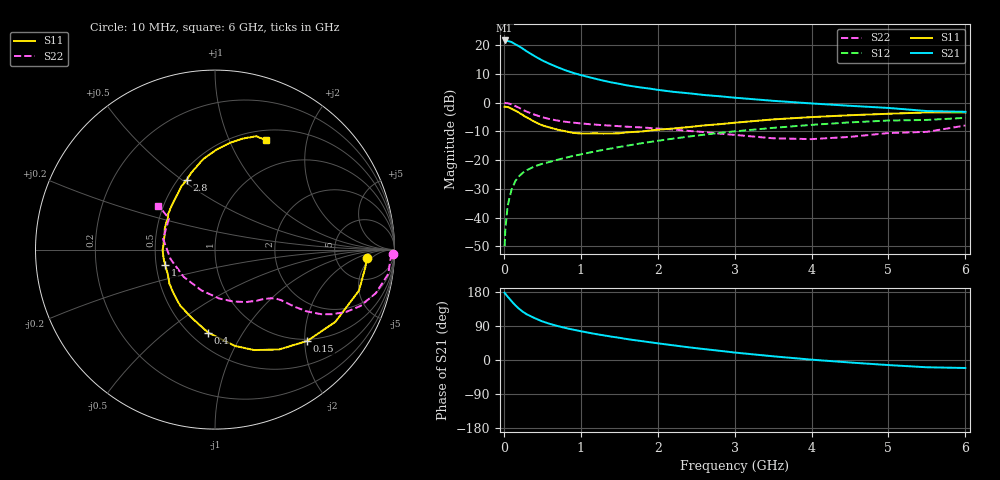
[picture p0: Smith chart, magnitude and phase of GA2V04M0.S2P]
! Infineon Technologies  Discrete & RF Semiconductors
! BF775
! Si NPN RF Bipolar Junction Transistor in SOT23
! VCE = 2 V  IC = 4 mA
! Common Emitter S-Parameters:  May  1996
# GHz  S  MA  R  50
!  f  S11  S21  S12  S22
! GHz  MAG  ANG  MAG  ANG  MAG  ANG  MAG  ANG
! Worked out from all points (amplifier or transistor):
!   36 points, 10 MHz to 6 GHz, reference 50 ohm
!   highest |S21| = 21.6 dB at 10 MHz (marker M1)
!   |S21| within 3 dB of that: start of sweep to 254.7 MHz
!   unconditionally stable (mu >= 1): 840.2 MHz to 4.023 GHz; 5.283 GHz to 5.9 GHz
!   at 250 MHz: K = 0.44, MSG = 21.5 dB, |S12| = -24.3 dB
!   at 1.4 GHz: K = 1.15, MAG = 9.1 dB, |S12| = -15.9 dB
!   at 6 GHz: K = 1.00, MSG = 1.1 dB, |S12| = -5.3 dB
!   S11 on the Smith chart (normalised r, x): 10 MHz: 11, -4; 150 MHz: 0.96, -2.06; 400 MHz: 0.61, -0.72; 1 GHz: 0.56, -0.11; 2.8 GHz: 0.55, +0.52; 6 GHz: 0.62, +1.38
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0.01  0.8474 -3.3  11.96 177.6  0.0032 88.6  0.9918 -1.5
0.02  0.844 -6.5  11.82 174.6  0.0064 90.0  0.9786 -3.2
0.05  0.8341 -15.9  11.71 167.2  0.0162 80.8  0.9749 -8.0
0.1  0.7821 -31.0  11.24 155.3  0.0307 73.6  0.9279 -15.2
0.15  0.7232 -44.7  10.26 144.1  0.0433 66.8  0.8692 -21.2
0.2  0.6613 -57.3  9.443 134.9  0.0527 62.3  0.808 -25.5
0.25  0.6008 -68.7  8.556 126.8  0.0608 58.1  0.7446 -28.9
0.3  0.5482 -78.3  7.698 120.4  0.067 56.1  0.6926 -31.3
0.4  0.464 -94.7  6.391 110.6  0.078 53.1  0.6155 -34.0
0.5  0.4009 -109.1  5.38 101.9  0.0862 51.7  0.5554 -35.4
0.6  0.3672 -122.0  4.664 95.2  0.0935 51.6  0.5139 -36.3
0.8  0.3172 -143.2  3.631 84.6  0.1095 51.7  0.4636 -37.4
1  0.2905 -162.6  3 76.0  0.1257 52.3  0.4338 -39.0
1.1  0.2907 -170.5  2.773 72.1  0.134 52.7  0.4222 -40.1
1.3  0.2883 174.8  2.388 65.0  0.1514 52.8  0.4032 -42.4
1.6  0.3036 157.1  1.986 55.3  0.1779 52.2  0.3801 -47.0
2.2  0.3538 130.6  1.535 38.8  0.2357 49.1  0.3401 -59.4
2.8  0.4199 111.8  1.286 24.4  0.2963 43.7  0.2883 -77.1
3.5  0.5089 97.4  1.071 9.8  0.3629 35.6  0.2392 -108.7
4.5  0.6016 81.9  0.877 -6.6  0.4518 22.5  0.2531 -167.9
5.5  0.6726 69.9  0.711 -19.2  0.4986 7.8  0.3095 145.9
6  0.6714 64.9  0.69 -21.1  0.5418 3.7  0.3993 142.1
